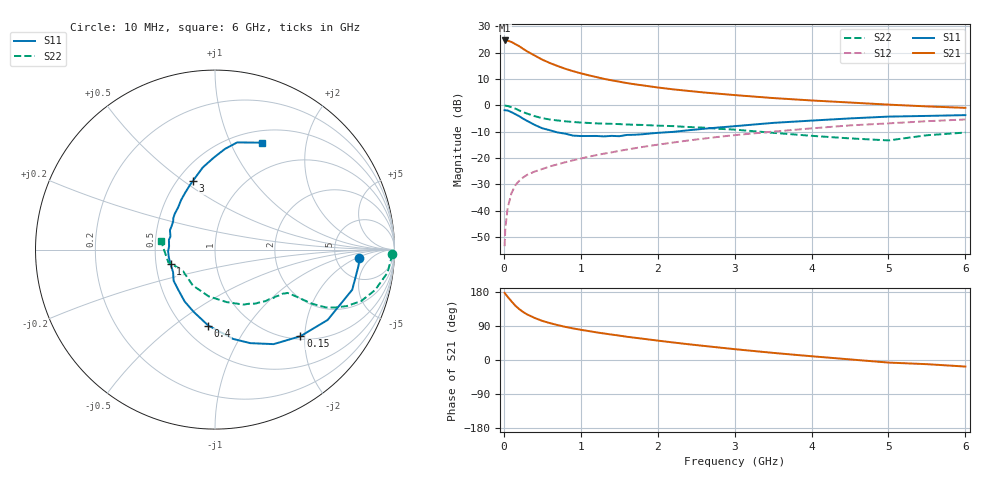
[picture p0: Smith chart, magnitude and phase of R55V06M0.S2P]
! SIEMENS Small Signal Semiconductors
! BFR183
! Si NPN RF Bipolar Junction Transistor in SOT23
! VCE = 5 V  IC = 6 mA
! Common Emitter S-Parameters:  May  1996
# GHz  S  MA  R  50
!  f  S11  S21  S12  S22
! GHz  MAG  ANG  MAG  ANG  MAG  ANG  MAG  ANG
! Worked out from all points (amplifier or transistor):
!   36 points, 10 MHz to 6 GHz, reference 50 ohm
!   highest |S21| = 24.7 dB at 10 MHz (marker M1)
!   |S21| within 3 dB of that: start of sweep to 241.3 MHz
!   unconditionally stable (mu >= 1): 962.3 MHz to 2.619 GHz
!   at 250 MHz: K = 0.47, MSG = 24.5 dB, |S12| = -27.5 dB
!   at 1.4 GHz: K = 1.06, MAG = 12.2 dB, |S12| = -17.9 dB
!   at 6 GHz: K = 0.88, MSG = 2.2 dB, |S12| = -5.4 dB
!   lowest NFmin = 1.20 dB at 450 MHz
!   S11 on the Smith chart (normalised r, x): 10 MHz: 8.67, -2.37; 150 MHz: 1.06, -1.90; 400 MHz: 0.65, -0.67; 1 GHz: 0.60, -0.11; 3 GHz: 0.60, +0.54; 6 GHz: 0.64, +1.32
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0.01  0.8063 -3.4  17.09 177.3  0.0021 91.5  0.987 -1.5
0.02  0.8045 -6.5  16.84 174.4  0.0047 84.6  0.9829 -3.0
0.05  0.7967 -16.3  16.91 166.7  0.0113 81.6  0.9698 -7.6
0.1  0.7399 -32.0  15.98 154.6  0.0215 74.1  0.9199 -14.2
0.15  0.6779 -45.4  14.54 143.3  0.0304 68.0  0.8631 -19.4
0.2  0.6197 -58.2  13.27 134.3  0.0366 64.8  0.7988 -23.2
0.25  0.5572 -69.3  11.86 126.8  0.0424 61.0  0.7414 -25.8
0.3  0.5084 -78.4  10.66 120.6  0.0475 60.2  0.6977 -27.5
0.4  0.4247 -95.1  8.843 111.0  0.055 57.9  0.6226 -29.1
0.5  0.3661 -109.1  7.383 103.2  0.0616 57.9  0.5689 -29.6
0.6  0.3349 -120.3  6.348 97.3  0.0691 57.9  0.5368 -29.9
0.8  0.2886 -143.0  4.938 87.4  0.0828 58.8  0.4961 -30.4
1  0.2604 -161.6  4.058 79.7  0.0973 60.3  0.4699 -30.9
1.1  0.2609 -170.3  3.731 76.4  0.1052 60.8  0.4621 -31.9
1.3  0.2565 175.9  3.19 70.1  0.1204 60.7  0.4484 -33.4
1.6  0.2732 156.7  2.646 61.3  0.1441 60.2  0.4323 -36.8
2.2  0.3125 131.0  2.012 46.3  0.196 57.5  0.4021 -45.6
3  0.401 108.1  1.564 28.6  0.2707 50.8  0.3451 -62.6
3.5  0.4632 98.4  1.374 18.8  0.316 45.2  0.2999 -77.4
4.5  0.5633 84.4  1.129 1.6  0.4148 33.4  0.2349 -121.8
5.5  0.6285 71.6  0.953 -11.0  0.4986 21.3  0.2697 -164.8
6  0.6507 66.3  0.894 -17.3  0.5382 13.3  0.3035 171.3
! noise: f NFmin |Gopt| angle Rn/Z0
0.45  1.2  0.21  41  0.24
0.9  1.25  0.24  101  0.21
1.8  2  0.32  175  0.14
